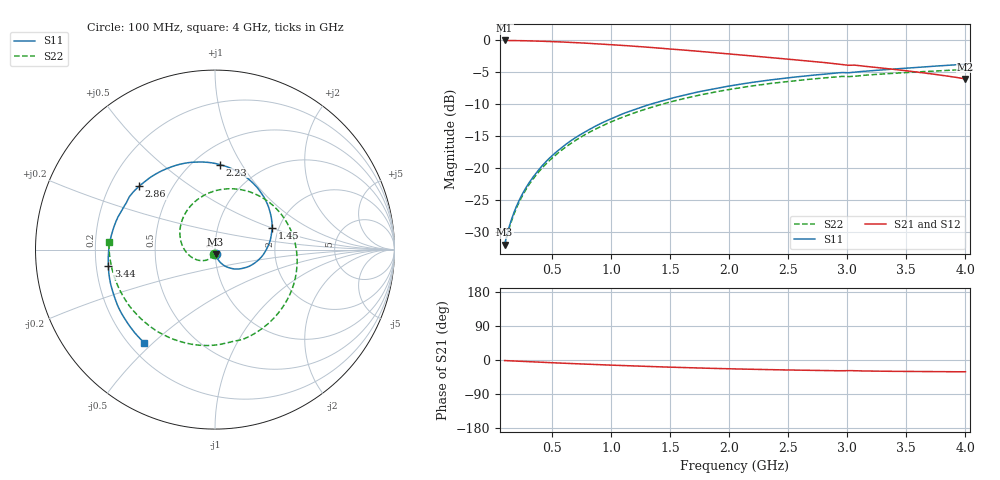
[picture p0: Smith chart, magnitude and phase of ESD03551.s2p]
! Created Thu Jun 14 15:57:09 2018
# hz S ma R 50
! 2 Port Network Data from SP1.SP block
! freq  magS11  angS11  magS21  angS21  magS12  angS12  magS22  angS22
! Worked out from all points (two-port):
!   391 points, 100 MHz to 4 GHz, reference 50 ohm
!   highest |S21| = -0.01 dB at 100 MHz (marker M1); lowest = -6.0 dB at 4 GHz (marker M2)
!   |S21| within 3 dB of the highest: start of sweep to 2.543 GHz
!   lowest |S11| = -31.9 dB at 100 MHz (marker M3), VSWR 1.05, Z = 50.3 - j2.52 ohm
!   |S11| at or under -10 dB: start of sweep to 1.33 GHz
!   |S22| runs from -32.2 to -4.5 dB; largest |S21 - S12| = 0.0039
!   S11 on the Smith chart (normalised r, x): 100 MHz: 1.01, -0.05; 1.45 GHz: 1.84, +0.51; 2.23 GHz: 0.66, +0.81; 2.86 GHz: 0.32, +0.33; 3.44 GHz: 0.25, -0.07; 4 GHz: 0.26, -0.47
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1e8  0.02528 -82.8  0.9989 -1.5  0.9992 -1.5  0.02464 -102.8
1.4e8  0.03528 -79.6  0.998 -2.1  0.9983 -2.0  0.03434 -107.8
1.9e8  0.04786 -76.0  0.9966 -2.8  0.9969 -2.8  0.04648 -114.1
3.1e8  0.07785 -67.3  0.9916 -4.5  0.992 -4.5  0.07547 -129.0
4.9e8  0.1227 -54.0  0.9796 -7.1  0.9808 -7.0  0.1175 -151.5
7.5e8  0.1853 -34.4  0.9558 -10.5  0.9571 -10.4  0.1766 176.8
1.08e9  0.2622 -8.9  0.916 -14.5  0.9184 -14.4  0.2473 137.3
1.4e9  0.33 16.9  0.8723 -17.9  0.8751 -17.8  0.3108 100.0
1.45e9  0.3403 21.0  0.8651 -18.4  0.8678 -18.3  0.3204 94.2
1.61e9  0.3711 34.3  0.8415 -19.9  0.8447 -19.9  0.3498 75.9
1.75e9  0.3976 46.0  0.8211 -21.2  0.8242 -21.1  0.3738 60.0
2.05e9  0.4476 71.3  0.777 -23.5  0.7802 -23.5  0.4203 26.5
2.23e9  0.4746 86.6  0.751 -24.8  0.7544 -24.7  0.4452 6.7
2.47e9  0.5068 107.1  0.7171 -26.2  0.7206 -26.2  0.4747 -19.5
2.7e9  0.5333 126.8  0.6857 -27.3  0.6891 -27.4  0.4988 -44.4
2.86e9  0.5506 140.2  0.6628 -28.1  0.6666 -28.1  0.5142 -61.7
3.13e9  0.5724 163.2  0.631 -28.9  0.6346 -29.0  0.5323 -90.3
3.35e9  0.5934 -178.5  0.6 -29.8  0.6035 -29.9  0.55 -114.0
3.44e9  0.6013 -171.2  0.5871 -30.1  0.5906 -30.2  0.5565 -123.7
3.58e9  0.6139 -159.9  0.5674 -30.5  0.5709 -30.6  0.5653 -138.6
3.75e9  0.6299 -146.3  0.5416 -30.9  0.5449 -31.0  0.5765 -157.0
4e9  0.6517 -127.1  0.5006 -31.0  0.5037 -31.2  0.5922 175.9
